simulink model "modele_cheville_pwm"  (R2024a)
settings: Solver=VariableStepAuto  StartTime=0.0  StopTime=0.5  RelTol=1e-3
InitFcn:
  | load_Tibia_gauche_leger_DataFile1
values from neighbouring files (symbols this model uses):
  smiData = saveVarsMat.smiData    [load_Tibia_gauche_leger_DataFile1.m]
undefined symbols (not defined in the file or in its folder): deg, kg, m, mm, N, s, X, Y, Z
libraries: fl_lib x19, sm_lib x16, nesl_utility x5, ee_lib x1

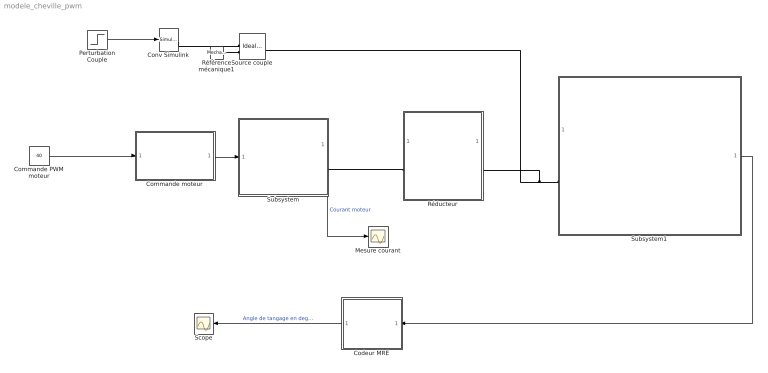
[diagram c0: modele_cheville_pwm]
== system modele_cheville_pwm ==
  Codeur MRE : Subsystem
  Commande PWM moteur : Constant  Value=40
  Commande moteur : Subsystem
  Conv Simulink : nesl_utility/Simulink-PS Converter  PhysicalDomain=network_engine_domain  SubClassName=ps_input  LeftPortType=input  RightPortType=output  PseudoPeriodic=off  Frequencies=[]  NoiseDistribution=none  NoiseParameters=[]  Unit=1  AffineConversion=off  FilteringAndDerivatives=zero  SimscapeFilterOrder=1  InputFilterTimeConstant=0.001  UdotUserProvided=1
  Mesure courant : Scope
  Perturbation Couple : Step  Time=0  After=-0.4*9.81*0.17  SampleTime=0
  Réducteur : Subsystem
  Référence mécanique1 : fl_lib/Mechanical/Rotational Elements/Mechanical Rotational Reference
  Scope : Scope
  Source couple : fl_lib/Mechanical/Mechanical Sources/Ideal Torque Source
  Subsystem : Subsystem
  Subsystem1 : Subsystem
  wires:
  Codeur MRE/1(Angle_de_tangage) -> Scope/1  "Angle de tangage en degré"
  Subsystem1/1(Position en degrés) -> Codeur MRE/1(In1)
  Subsystem/1(Courant moteur) -> Mesure courant/1  "Courant moteur"
  Commande moteur/1(Out1) -> Subsystem/1(input0)
  Perturbation Couple/1 -> Conv Simulink/1
  Commande PWM moteur/1 -> Commande moteur/1(In1)
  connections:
  Réducteur/LConn1 -- Subsystem/RConn1
  Subsystem1/LConn1 -- Source couple/LConn1 -- Réducteur/RConn1
  Conv Simulink/RConn1 -- Source couple/RConn1
  Référence mécanique1/LConn1 -- Source couple/RConn2

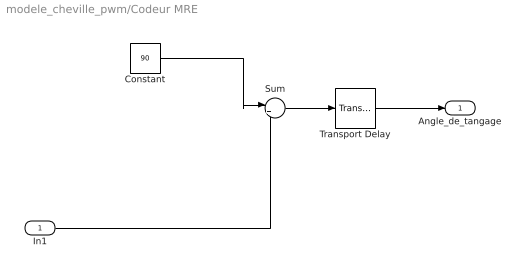
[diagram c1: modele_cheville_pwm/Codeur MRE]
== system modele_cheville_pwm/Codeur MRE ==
  In1 : Inport
  Constant : Constant  Value=90
  Sum : Sum  Inputs=|++
  Transport Delay : TransportDelay  DelayTime=1E-2
  Angle_de_tangage : Outport
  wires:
  Constant/1 -> Sum/1
  In1/1 -> Sum/2
  Sum/1 -> Transport Delay/1
  Transport Delay/1 -> Angle_de_tangage/1

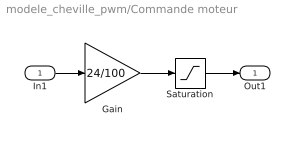
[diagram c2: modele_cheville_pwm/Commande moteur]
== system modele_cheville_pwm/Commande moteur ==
  In1 : Inport
  Gain : Gain  Gain=24/100
  Saturation : Saturate  UpperLimit=24  LowerLimit=-24
  Out1 : Outport
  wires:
  Gain/1 -> Saturation/1
  Saturation/1 -> Out1/1
  In1/1 -> Gain/1

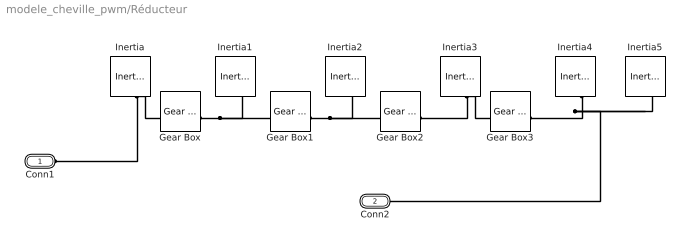
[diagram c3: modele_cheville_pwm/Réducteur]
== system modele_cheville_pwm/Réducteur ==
  Gear Box : fl_lib/Mechanical/Mechanisms/Gear Box  ratio=4  t_in_specify=off  t_in_priority=None  t_in=0 N*m  t_in_nominal_specify=off  t_in_nominal_value=1  t_in_nominal_unit=N*m  t_out_specify=off  t_out_priority=None  t_out=0 N*m  t_out_nominal_specify=off  t_out_nominal_value=1  t_out_nominal_unit=N*m
  Gear Box1 : fl_lib/Mechanical/Mechanisms/Gear Box  ratio=1.88  t_in_specify=off  t_in_priority=None  t_in=0 N*m  t_in_nominal_specify=off  t_in_nominal_value=1  t_in_nominal_unit=N*m  t_out_specify=off  t_out_priority=None  t_out=0 N*m  t_out_nominal_specify=off  t_out_nominal_value=1  t_out_nominal_unit=N*m
  Gear Box2 : fl_lib/Mechanical/Mechanisms/Gear Box  ratio=4.83  t_in_specify=off  t_in_priority=None  t_in=0 N*m  t_in_nominal_specify=off  t_in_nominal_value=1  t_in_nominal_unit=N*m  t_out_specify=off  t_out_priority=None  t_out=0 N*m  t_out_nominal_specify=off  t_out_nominal_value=1  t_out_nominal_unit=N*m
  Gear Box3 : fl_lib/Mechanical/Mechanisms/Gear Box  ratio=3.6  t_in_specify=off  t_in_priority=None  t_in=0 N*m  t_in_nominal_specify=off  t_in_nominal_value=1  t_in_nominal_unit=N*m  t_out_specify=off  t_out_priority=None  t_out=0 N*m  t_out_nominal_specify=off  t_out_nominal_value=1  t_out_nominal_unit=N*m
  Inertia : fl_lib/Mechanical/Rotational Elements/Inertia  inertia=4.8e2 g*mm^2  num_ports=foundation.enum.numPorts2.one  w_specify=off  w_priority=None  w=0 rad/s  w_nominal_specify=off  w_nominal_value=1  w_nominal_unit=rad/s  t_specify=off  t_priority=None  t=0 N*m  t_nominal_specify=off  t_nominal_value=1  t_nominal_unit=N*m
  Inertia1 : fl_lib/Mechanical/Rotational Elements/Inertia  inertia=4.7 mm^2*g  num_ports=foundation.enum.numPorts2.one  w_specify=off  w_priority=None  w=0 rad/s  w_nominal_specify=off  w_nominal_value=1  w_nominal_unit=rad/s  t_specify=off  t_priority=None  t=0 N*m  t_nominal_specify=off  t_nominal_value=1  t_nominal_unit=N*m
  Inertia2 : fl_lib/Mechanical/Rotational Elements/Inertia  inertia=80 mm^2*g  num_ports=foundation.enum.numPorts2.one  w_specify=off  w_priority=None  w=0 rad/s  w_nominal_specify=off  w_nominal_value=1  w_nominal_unit=rad/s  t_specify=off  t_priority=None  t=0 N*m  t_nominal_specify=off  t_nominal_value=1  t_nominal_unit=N*m
  Inertia3 : fl_lib/Mechanical/Rotational Elements/Inertia  inertia=30 mm^2*g  num_ports=foundation.enum.numPorts2.one  w_specify=off  w_priority=None  w=0 rad/s  w_nominal_specify=off  w_nominal_value=1  w_nominal_unit=rad/s  t_specify=off  t_priority=None  t=0 N*m  t_nominal_specify=off  t_nominal_value=1  t_nominal_unit=N*m
  Inertia4 : fl_lib/Mechanical/Rotational Elements/Inertia  inertia=1095 mm^2*g  num_ports=foundation.enum.numPorts2.one  w_specify=off  w_priority=None  w=0 rad/s  w_nominal_specify=off  w_nominal_value=1  w_nominal_unit=rad/s  t_specify=off  t_priority=None  t=0 N*m  t_nominal_specify=off  t_nominal_value=1  t_nominal_unit=N*m
  Inertia5 : fl_lib/Mechanical/Rotational Elements/Inertia  inertia=2.6e6 mm^2*g  num_ports=foundation.enum.numPorts2.one  w_specify=off  w_priority=None  w=0 rad/s  w_nominal_specify=off  w_nominal_value=1  w_nominal_unit=rad/s  t_specify=off  t_priority=None  t=0 N*m  t_nominal_specify=off  t_nominal_value=1  t_nominal_unit=N*m
  Conn1 : PMIOPort  Side=Left
  Conn2 : PMIOPort  Port=2  Side=Right
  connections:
  Gear Box1/RConn1 -- Gear Box2/LConn1 -- Inertia2/LConn1
  Inertia/LConn1 -- Conn1/RConn1 -- Gear Box/LConn1
  Inertia3/LConn1 -- Gear Box3/LConn1 -- Gear Box2/RConn1
  Inertia4/LConn1 -- Conn2/RConn1 -- Inertia5/LConn1 -- Gear Box3/RConn1
  Gear Box/RConn1 -- Inertia1/LConn1 -- Gear Box1/LConn1

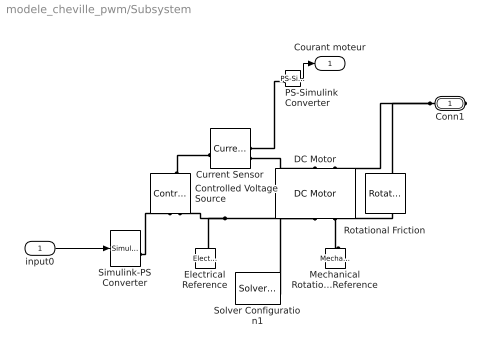
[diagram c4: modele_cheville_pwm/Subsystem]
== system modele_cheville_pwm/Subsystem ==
  input0 : Inport
  Controlled Voltage Source : fl_lib/Electrical/Electrical Sources/Controlled Voltage Source
  Current Sensor : fl_lib/Electrical/Electrical Sensors/Current Sensor
  DC Motor : ee_lib/Electromechanical/Brushed Motors/DC Motor  field_option=ee.enum.field_option.pm  Rf=100 Ohm  Lf=1 H  Laf=0.15 H  If0=0 A  parameterization=1  Ra=5.4 Ohm  La=0.6 mH  emf_or_torque=1  Kv=19.6e-3 V/(rad/s)  Ki=6.876e-4 N*m/A  T_stall=2.4e-4 N*m  w_max=1.91e+4 rpm  w_rated=1.5e+4 rpm  P_rated=0.08 W  V_rated=1.5 V  lam_param=1  i_noload=0 A  V_i_noload=1.5 V  J=0.01 g*cm^2  lam=0 N*m/(rad/s)  speed0=0 rpm  enable_fault_armature=simscape.enum.onoff.off  rev_faulted=1 / 3  G_faulted_armature=1e-5 S  fault_trigger_armature=ee.enum.faults.faultTrigger.temporal  t_fault_armature=1 s  max_permissible_current_armature=inf A  t_fail_on_current_armature=1 s  enable_fault_field=simscape.enum.onoff.off  G_faulted_field=1e-5 S  fault_trigger_field=ee.enum.faults.faultTrigger.temporal  t_fault_field=1 s  max_permissible_current_field=inf A  t_fail_on_current_field=1 s  fault_action=simscape.enum.assert.action.none  alpha=3.93e-3 1/K  Tmeas=25 degC  thermal_mass=100 J/K  initial_temperature=25 degC
  Electrical Reference : fl_lib/Electrical/Electrical Elements/Electrical Reference
  Mechanical Rotational Reference : fl_lib/Mechanical/Rotational Elements/Mechanical Rotational Reference
  PS-Simulink Converter : nesl_utility/PS-Simulink Converter  PhysicalDomain=network_engine_domain  SubClassName=ps_output  LeftPortType=input  RightPortType=output  PseudoPeriodic=off  Frequencies=[]  VectorFormat=inherit  Unit=inherit  AffineConversion=off
  Rotational Friction : fl_lib/Mechanical/Rotational Elements/Rotational Friction  brkwy_trq=8 mN*m  brkwy_vel=0.0060623 rad/s  Col_trq=8 mN*m  visc_coef=0 N*m/(rad/s)  w_specify=off  w_priority=High  w=0 rad/s  w_nominal_specify=off  w_nominal_value=1  w_nominal_unit=rad/s  t_specify=off  t_priority=High  t=0 N*m  t_nominal_specify=off  t_nominal_value=1  t_nominal_unit=N*m
  Simulink-PS Converter : nesl_utility/Simulink-PS Converter  PhysicalDomain=network_engine_domain  SubClassName=ps_input  LeftPortType=input  RightPortType=output  PseudoPeriodic=off  Frequencies=[]  NoiseDistribution=none  NoiseParameters=[]  Unit=1  AffineConversion=off  FilteringAndDerivatives=zero  SimscapeFilterOrder=1  InputFilterTimeConstant=0.001  UdotUserProvided=1
  Solver Configuration1 : nesl_utility/Solver Configuration  PhysicalDomain=network_engine_domain  SubClassName=solver  LeftPortType=input  RightPortType=generic  Tones=[]  Harmonics=[]  SimulateNoise=off  Profile=off  UseLocalSampling=off  EnableSwitchedLinearOptims=on  FrequencyDomain=off  UseCCode=off  RelTol=0.001  AbsTol=1e-06  MinStep=1e-09  ToWorkspace=off  RevertToSquareIcSolve=off  NumHomotopyIterations=100  PhasorMode=off  PhasorModeNumHarmonics=1  ConsistencySolver=NEWTON_FTOL  IndexReductionMethod=DerivativeReplacement  DoDC=off  ResidualTolerance=1e-6  ConsistencyTolSource=GLOBAL  ConsistencyAbsTol=0.001  ConsistencyRelTol=0.001  ConsistencyTolFactor=0.001  UseLocalSolver=off  LocalSolverChoice=NE_BACKWARD_EULER_ADVANCER  ResolveIndetEquations=on  FunctionEvalNumThread=1  LocalSolverSampleTime=0.001  DoFixedCost=on  MaxNonlinIter=100  MaxModeIter=10  ComputeImpulses=off  ImpulseIterations=2  LinearAlgebra=Sparse  LinearAlgebraNumThread=0  EquationFormulation=NE_TIME_EF  DelaysMemoryBudget=1024  AutomaticFiltering=on  FilteringTimeConstant=0.001  PartitionStorageMethod=AS_NEEDED  PartitionMemoryBudget=1024  PartitionMethod=FAST  MultibodyUseLocalSolver=off  MultibodyLocalSolverChoice=ODE1  MultibodyLocalSolverSampleTime=0.001
  Conn1 : PMIOPort  Side=Right
  Courant moteur : Outport
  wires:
  PS-Simulink Converter/1 -> Courant moteur/1
  input0/1 -> Simulink-PS Converter/1
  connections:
  PS-Simulink Converter/LConn1 -- Current Sensor/RConn1
  Conn1/RConn1 -- Rotational Friction/LConn1 -- DC Motor/LConn2
  DC Motor/RConn1 -- Electrical Reference/LConn1 -- Controlled Voltage Source/RConn2 -- Solver Configuration1/RConn1
  DC Motor/RConn2 -- Rotational Friction/RConn1 -- Mechanical Rotational Reference/LConn1
  Simulink-PS Converter/RConn1 -- Controlled Voltage Source/RConn1
  Controlled Voltage Source/LConn1 -- Current Sensor/LConn1
  Current Sensor/RConn2 -- DC Motor/LConn1

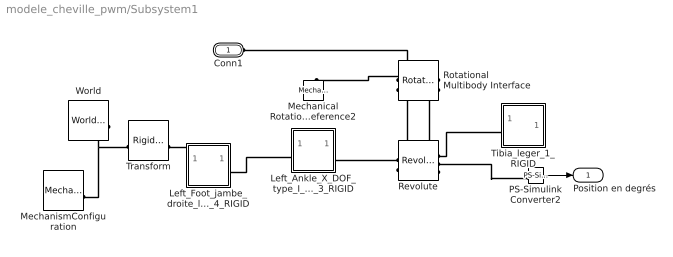
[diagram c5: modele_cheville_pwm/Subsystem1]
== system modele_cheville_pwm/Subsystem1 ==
  Left_Ankle_X_DOF_type_I_leger_3_RIGID : Subsystem
  Left_Foot_jambe_droite_leger_4_RIGID : Subsystem
  Mechanical Rotational Reference2 : fl_lib/Mechanical/Rotational Elements/Mechanical Rotational Reference
  MechanismConfiguration : sm_lib/Utilities/Mechanism Configuration  UniformGravity=Constant  GravityVector=[0 -9.80665 0]  GravityVectorUnits=m/s^2  LinearizationDelta=0.001  JointModeTransitionNonlinearIterations=2
  PS-Simulink Converter2 : nesl_utility/PS-Simulink Converter  PhysicalDomain=network_engine_domain  SubClassName=ps_output  LeftPortType=input  RightPortType=output  PseudoPeriodic=off  Frequencies=[]  VectorFormat=inherit  Unit=deg  AffineConversion=off
  Revolute : sm_lib/Joints/Revolute Joint  JointMode=Normal  CompositeWrenchDir=FollowerOnBase  CompositeWrenchFrame=BaseFrame  SenseConstraintForce=off  SenseConstraintTorque=off  SenseTotalForce=off  SenseTotalTorque=off  PositionTargetSpecify=on  PositionTargetPriority=Low  PositionTargetValue=smiData.RevoluteJoint(1).Rz.Pos  PositionTargetValueUnits=deg  VelocityTargetSpecify=off  VelocityTargetPriority=High  VelocityTargetValue=0  VelocityTargetValueUnits=deg/s  EquilibriumPosition=0  EquilibriumPositionUnits=deg  SpringStiffness=0  SpringStiffnessUnits=N*m/deg  DampingCoefficient=0  DampingCoefficientUnits=N*m/(deg/s)  LowerLimitSpecify=off  LowerLimitBound=-90  LowerLimitBoundUnits=deg  LowerLimitStiffness=1e4  LowerLimitStiffnessUnits=N*m/deg  LowerLimitDamping=10  LowerLimitDampingUnits=N*m/(deg/s)  LowerLimitTransitionRegionWidth=0.1  LowerLimitTransitionRegionWidthUnits=deg  UpperLimitSpecify=off  UpperLimitBound=90  UpperLimitBoundUnits=deg  UpperLimitStiffness=1e4  UpperLimitStiffnessUnits=N*m/deg  UpperLimitDamping=10  UpperLimitDampingUnits=N*m/(deg/s)  UpperLimitTransitionRegionWidth=0.1  UpperLimitTransitionRegionWidthUnits=deg  TorqueActuationMode=InputTorque  MotionActuationMode=ComputedMotion  SensePosition=on  SenseVelocity=on  SenseAcceleration=off  SenseTorqueForce=off  SenseLowerLimitTorqueForce=off  SenseUpperLimitTorqueForce=off
  Rotational Multibody Interface : fl_lib/Mechanical/Multibody Interfaces/Rotational Multibody Interface
  Tibia_leger_1_RIGID : Subsystem
  Transform : sm_lib/Frames and Transforms/Rigid Transform  RotationMethod=ArbitraryAxis  FollAlignAxisA=+X  BaseAlignAxisA=+Y  FollAlignAxisB=+Y  BaseAlignAxisB=+Z  RotationStandardAxis=+Z  RotationAngle=smiData.RigidTransform(5).angle  RotationAngleUnits=rad  RotationArbitraryAxis=smiData.RigidTransform(5).axis  RotationSequenceAxes=FollowerAxes  RotationSequence=XYX  RotationSequenceAngles=[0 0 0]  RotationSequenceAnglesUnits=deg  RotationMatrix=[1 0 0; 0 1 0; 0 0 1]  Quaternion=[1 0 0 0]  TranslationMethod=Cartesian  TranslationCartesianOffset=smiData.RigidTransform(5).translation  TranslationCartesianOffsetUnits=mm  TranslationStandardAxis=+Z  TranslationStandardOffset=0  TranslationStandardOffsetUnits=mm  TranslationROffset=0  TranslationROffsetUnits=m  TranslationThetaOffset=0  TranslationThetaOffsetUnits=deg  TranslationZOffset=0  TranslationZOffsetUnits=m
  World : sm_lib/Frames and Transforms/World Frame
  Conn1 : PMIOPort  Side=Left
  Position en degrés : Outport
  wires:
  PS-Simulink Converter2/1 -> Position en degrés/1
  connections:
  Rotational Multibody Interface/RConn2 -- Conn1/RConn1
  Revolute/RConn1 -- Tibia_leger_1_RIGID/LConn1
  Rotational Multibody Interface/LConn2 -- Mechanical Rotational Reference2/LConn1
  MechanismConfiguration/RConn1 -- Transform/LConn1 -- World/RConn1
  Rotational Multibody Interface/RConn1 -- Revolute/RConn3
  Left_Foot_jambe_droite_leger_4_RIGID/LConn1 -- Transform/RConn1
  Left_Foot_jambe_droite_leger_4_RIGID/RConn1 -- Left_Ankle_X_DOF_type_I_leger_3_RIGID/LConn1
  Left_Ankle_X_DOF_type_I_leger_3_RIGID/RConn1 -- Revolute/LConn1
  Rotational Multibody Interface/LConn1 -- Revolute/LConn2
  Revolute/RConn2 -- PS-Simulink Converter2/LConn1

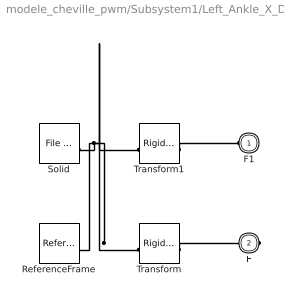
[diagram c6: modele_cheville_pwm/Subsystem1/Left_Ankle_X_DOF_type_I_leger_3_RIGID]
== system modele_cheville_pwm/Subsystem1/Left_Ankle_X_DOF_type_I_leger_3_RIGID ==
  ReferenceFrame : sm_lib/Frames and Transforms/Reference Frame
  Solid : sm_lib/Body Elements/File Solid  ExtGeomFileName=Left_Ankle_X_DOF_type I_leger_Default_sldprt.STEP  UnitType=FromFile  ExtGeomFileUnits=m  StepReaderType=HEX  ExportConvexHullGeometry=off  InertiaType=Custom  BasedOnType=DensityFromFile  Density=1000  DensityUnits=kg/m^3  Mass=smiData.Solid(2).mass  MassUnits=kg  CenterOfMass=smiData.Solid(2).CoM  CenterOfMassUnits=mm  MomentsOfInertia=smiData.Solid(2).MoI  MomentsOfInertiaUnits=kg*mm^2  ProductsOfInertia=smiData.Solid(2).PoI  ProductsOfInertiaUnits=kg*mm^2  GraphicType=FromGeometry  MarkerShape=Sphere  MarkerSize=10  GraphicVisPropType=SimpleVisualProperties  GraphicDiffuseColor=smiData.Solid(2).color  GraphicOpacity=smiData.Solid(2).opacity  GraphicSpecularColor=[0.5 0.5 0.5 1.0]  GraphicAmbientColor=[0.15 0.15 0.15 1.0]  GraphicEmissiveColor=[0.0 0.0 0.0 1.0]  GraphicShininess=75  DoExposeReferenceFrame=on  SerializedFrames=<Frames/>
  Transform : sm_lib/Frames and Transforms/Rigid Transform  RotationMethod=ArbitraryAxis  FollAlignAxisA=+X  BaseAlignAxisA=+Y  FollAlignAxisB=+Y  BaseAlignAxisB=+Z  RotationStandardAxis=+Z  RotationAngle=smiData.RigidTransform(1).angle  RotationAngleUnits=rad  RotationArbitraryAxis=smiData.RigidTransform(1).axis  RotationSequenceAxes=FollowerAxes  RotationSequence=XYX  RotationSequenceAngles=[0 0 0]  RotationSequenceAnglesUnits=deg  RotationMatrix=[1 0 0; 0 1 0; 0 0 1]  Quaternion=[1 0 0 0]  TranslationMethod=Cartesian  TranslationCartesianOffset=smiData.RigidTransform(1).translation  TranslationCartesianOffsetUnits=mm  TranslationStandardAxis=+Z  TranslationStandardOffset=0  TranslationStandardOffsetUnits=mm  TranslationROffset=0  TranslationROffsetUnits=m  TranslationThetaOffset=0  TranslationThetaOffsetUnits=deg  TranslationZOffset=0  TranslationZOffsetUnits=m
  Transform1 : sm_lib/Frames and Transforms/Rigid Transform  RotationMethod=ArbitraryAxis  FollAlignAxisA=+X  BaseAlignAxisA=+Y  FollAlignAxisB=+Y  BaseAlignAxisB=+Z  RotationStandardAxis=+Z  RotationAngle=smiData.RigidTransform(4).angle  RotationAngleUnits=rad  RotationArbitraryAxis=smiData.RigidTransform(4).axis  RotationSequenceAxes=FollowerAxes  RotationSequence=XYX  RotationSequenceAngles=[0 0 0]  RotationSequenceAnglesUnits=deg  RotationMatrix=[1 0 0; 0 1 0; 0 0 1]  Quaternion=[1 0 0 0]  TranslationMethod=Cartesian  TranslationCartesianOffset=smiData.RigidTransform(4).translation  TranslationCartesianOffsetUnits=mm  TranslationStandardAxis=+Z  TranslationStandardOffset=0  TranslationStandardOffsetUnits=mm  TranslationROffset=0  TranslationROffsetUnits=m  TranslationThetaOffset=0  TranslationThetaOffsetUnits=deg  TranslationZOffset=0  TranslationZOffsetUnits=m
  F1 : PMIOPort  Side=Left
  F : PMIOPort  Port=2  Side=Right
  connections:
  Solid/RConn1 -- ReferenceFrame/RConn1 -- Transform/LConn1 -- Transform1/LConn1
  Transform/RConn1 -- F/RConn1
  Transform1/RConn1 -- F1/RConn1

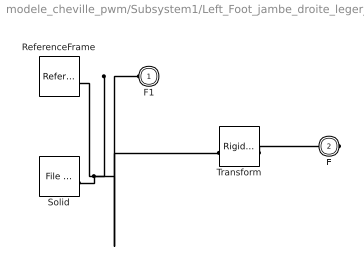
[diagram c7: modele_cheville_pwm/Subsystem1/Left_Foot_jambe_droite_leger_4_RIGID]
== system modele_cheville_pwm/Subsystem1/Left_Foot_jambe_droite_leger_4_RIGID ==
  ReferenceFrame : sm_lib/Frames and Transforms/Reference Frame
  Solid : sm_lib/Body Elements/File Solid  ExtGeomFileName=Left_Foot_jambe droite_leger_Default_sldprt.STEP  UnitType=FromFile  ExtGeomFileUnits=m  StepReaderType=HEX  ExportConvexHullGeometry=off  InertiaType=Custom  BasedOnType=DensityFromFile  Density=1000  DensityUnits=kg/m^3  Mass=smiData.Solid(3).mass  MassUnits=kg  CenterOfMass=smiData.Solid(3).CoM  CenterOfMassUnits=mm  MomentsOfInertia=smiData.Solid(3).MoI  MomentsOfInertiaUnits=kg*mm^2  ProductsOfInertia=smiData.Solid(3).PoI  ProductsOfInertiaUnits=kg*mm^2  GraphicType=FromGeometry  MarkerShape=Sphere  MarkerSize=10  GraphicVisPropType=SimpleVisualProperties  GraphicDiffuseColor=smiData.Solid(3).color  GraphicOpacity=smiData.Solid(3).opacity  GraphicSpecularColor=[0.5 0.5 0.5 1.0]  GraphicAmbientColor=[0.15 0.15 0.15 1.0]  GraphicEmissiveColor=[0.0 0.0 0.0 1.0]  GraphicShininess=75  DoExposeReferenceFrame=on  SerializedFrames=<Frames/>
  Transform : sm_lib/Frames and Transforms/Rigid Transform  RotationMethod=ArbitraryAxis  FollAlignAxisA=+X  BaseAlignAxisA=+Y  FollAlignAxisB=+Y  BaseAlignAxisB=+Z  RotationStandardAxis=+Z  RotationAngle=smiData.RigidTransform(3).angle  RotationAngleUnits=rad  RotationArbitraryAxis=smiData.RigidTransform(3).axis  RotationSequenceAxes=FollowerAxes  RotationSequence=XYX  RotationSequenceAngles=[0 0 0]  RotationSequenceAnglesUnits=deg  RotationMatrix=[1 0 0; 0 1 0; 0 0 1]  Quaternion=[1 0 0 0]  TranslationMethod=Cartesian  TranslationCartesianOffset=smiData.RigidTransform(3).translation  TranslationCartesianOffsetUnits=mm  TranslationStandardAxis=+Z  TranslationStandardOffset=0  TranslationStandardOffsetUnits=mm  TranslationROffset=0  TranslationROffsetUnits=m  TranslationThetaOffset=0  TranslationThetaOffsetUnits=deg  TranslationZOffset=0  TranslationZOffsetUnits=m
  F1 : PMIOPort  Side=Left
  F : PMIOPort  Port=2  Side=Right
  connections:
  Solid/RConn1 -- ReferenceFrame/RConn1 -- Transform/LConn1 -- F1/RConn1
  Transform/RConn1 -- F/RConn1

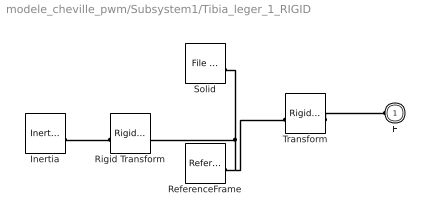
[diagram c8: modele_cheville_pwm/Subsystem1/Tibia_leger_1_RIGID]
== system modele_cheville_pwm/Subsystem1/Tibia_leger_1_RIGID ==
  Inertia : sm_lib/Body Elements/Inertia  Commented=on  InertiaType=PointMass  Mass=2.25  MassUnits=kg  CenterOfMass=[0 0 0]  CenterOfMassUnits=m  MomentsOfInertia=[1 1 1]  MomentsOfInertiaUnits=kg*m^2  ProductsOfInertia=[0 0 0]  ProductsOfInertiaUnits=kg*m^2  GraphicType=Marker  MarkerShape=Sphere  MarkerSize=50  GraphicVisPropType=AdvancedVisualProperties  GraphicDiffuseColor=[0.5 0.5 0.5]  GraphicOpacity=1  GraphicSpecularColor=[0.5 0.5 0.5 1.0]  GraphicAmbientColor=[0.15 0.15 0.15 1.0]  GraphicEmissiveColor=[0.0 0.0 0.0 1.0]  GraphicShininess=75
  ReferenceFrame : sm_lib/Frames and Transforms/Reference Frame
  Rigid Transform : sm_lib/Frames and Transforms/Rigid Transform  Commented=on  RotationMethod=None  FollAlignAxisA=+X  BaseAlignAxisA=+Y  FollAlignAxisB=+Y  BaseAlignAxisB=+Z  RotationStandardAxis=+Z  RotationAngle=0  RotationAngleUnits=deg  RotationArbitraryAxis=[0 0 1]  RotationSequenceAxes=FollowerAxes  RotationSequence=XYX  RotationSequenceAngles=[0 0 0]  RotationSequenceAnglesUnits=deg  RotationMatrix=[1 0 0;0 1 0;0 0 1]  Quaternion=[1 0 0 0]  TranslationMethod=Cartesian  TranslationCartesianOffset=[0 -0.3 0]  TranslationCartesianOffsetUnits=m  TranslationStandardAxis=+Z  TranslationStandardOffset=0  TranslationStandardOffsetUnits=m  TranslationROffset=0  TranslationROffsetUnits=m  TranslationThetaOffset=0  TranslationThetaOffsetUnits=deg  TranslationZOffset=0  TranslationZOffsetUnits=m
  Solid : sm_lib/Body Elements/File Solid  ExtGeomFileName=Tibia_leger_Default_sldprt.STEP  UnitType=FromFile  ExtGeomFileUnits=m  StepReaderType=HEX  ExportConvexHullGeometry=off  InertiaType=Custom  BasedOnType=DensityFromFile  Density=1000  DensityUnits=kg/m^3  Mass=smiData.Solid(1).mass  MassUnits=kg  CenterOfMass=smiData.Solid(1).CoM  CenterOfMassUnits=mm  MomentsOfInertia=smiData.Solid(1).MoI  MomentsOfInertiaUnits=kg*mm^2  ProductsOfInertia=smiData.Solid(1).PoI  ProductsOfInertiaUnits=kg*mm^2  GraphicType=FromGeometry  MarkerShape=Sphere  MarkerSize=10  GraphicVisPropType=SimpleVisualProperties  GraphicDiffuseColor=smiData.Solid(1).color  GraphicOpacity=smiData.Solid(1).opacity  GraphicSpecularColor=[0.5 0.5 0.5 1.0]  GraphicAmbientColor=[0.15 0.15 0.15 1.0]  GraphicEmissiveColor=[0.0 0.0 0.0 1.0]  GraphicShininess=75  DoExposeReferenceFrame=on  SerializedFrames=<Frames/>
  Transform : sm_lib/Frames and Transforms/Rigid Transform  RotationMethod=ArbitraryAxis  FollAlignAxisA=+X  BaseAlignAxisA=+Y  FollAlignAxisB=+Y  BaseAlignAxisB=+Z  RotationStandardAxis=+Z  RotationAngle=smiData.RigidTransform(2).angle  RotationAngleUnits=rad  RotationArbitraryAxis=smiData.RigidTransform(2).axis  RotationSequenceAxes=FollowerAxes  RotationSequence=XYX  RotationSequenceAngles=[0 0 0]  RotationSequenceAnglesUnits=deg  RotationMatrix=[1 0 0; 0 1 0; 0 0 1]  Quaternion=[1 0 0 0]  TranslationMethod=Cartesian  TranslationCartesianOffset=smiData.RigidTransform(2).translation  TranslationCartesianOffsetUnits=mm  TranslationStandardAxis=+Z  TranslationStandardOffset=0  TranslationStandardOffsetUnits=mm  TranslationROffset=0  TranslationROffsetUnits=m  TranslationThetaOffset=0  TranslationThetaOffsetUnits=deg  TranslationZOffset=0  TranslationZOffsetUnits=m
  F : PMIOPort  Side=Left
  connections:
  ReferenceFrame/RConn1 -- Transform/LConn1 -- Solid/RConn1 -- Rigid Transform/RConn1
  Transform/RConn1 -- F/RConn1
  Inertia/RConn1 -- Rigid Transform/LConn1
